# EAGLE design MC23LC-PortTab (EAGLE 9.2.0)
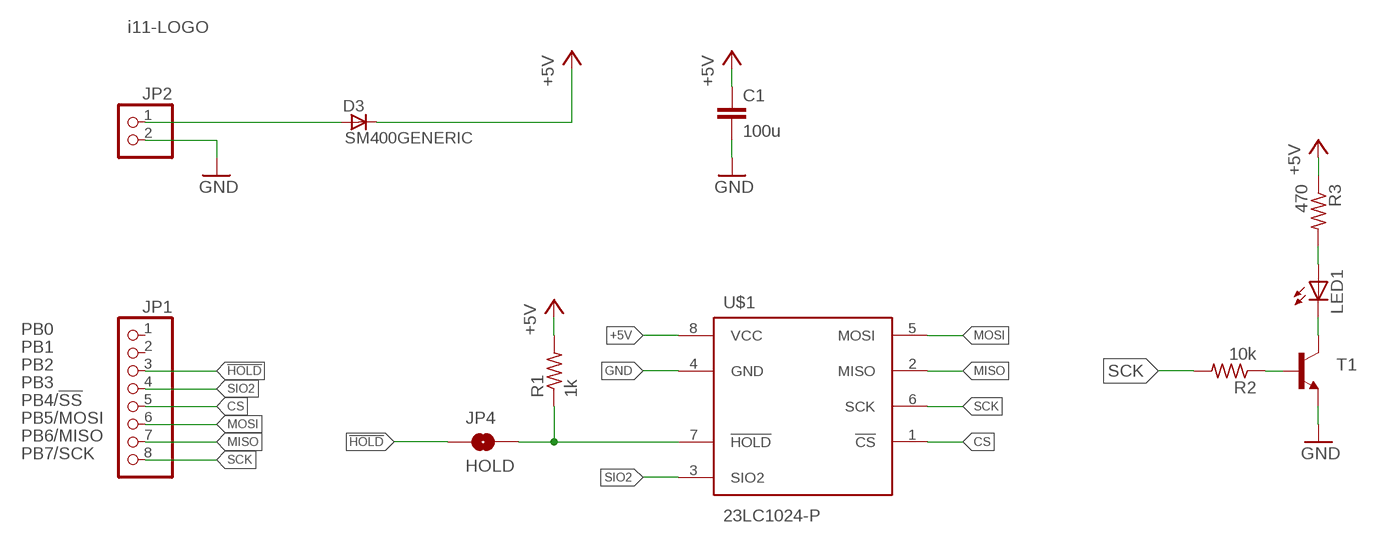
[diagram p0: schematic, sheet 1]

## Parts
C1  100u  C-EUC1206  [C1206]
D3  SM400GENERIC  [MELF-MLL41_DO213AB]
JP1  PINHD-1X8  [1X08]
JP2  PINHD-1X2  [1X02]
JP4  HOLD  JUMPER-SMT_2_NO_SILK  [SMT-JUMPER_2_NO_SILK]
LED1  LEDCHIPLED_1206  [CHIPLED_1206]
R1  1k  R-US_R1206  [R1206]
R2  10k  R-US_R1206  [R1206]
R3  470  R-US_R1206  [R1206]
T1  BC817-16-NPN-SOT23-BEC  [SOT23-BEC]
U$1  23LC1024-P  [DIL8]

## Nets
!HOLD!: JP1.3 JP4.1
+5V: C1.1 D3.C R1.2 R3.1 U$1.8(VCC)
CS: JP1.5 U$1.1(!CS!)
GND: C1.2 JP2.2 T1.E U$1.4(GND)
MISO: JP1.7 U$1.2(MISO)
MOSI: JP1.6 U$1.5(MOSI)
N$1: D3.A JP2.1
N$2: JP4.2 R1.1 U$1.7(!HOLD!)
N$3: R2.1 T1.B
N$5: LED1.C T1.C
N$6: LED1.A R3.2
SCK: JP1.8 R2.2 U$1.6(SCK)
SIO2: JP1.4 U$1.3(SIO2)
Unconnected: JP1.1 JP1.2

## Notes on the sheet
- i11-LOGO
- PB0
- PB1
- PB2
- PB3
- PB4/!SS!
- PB5/MOSI
- PB6/MISO
- PB7/SCK

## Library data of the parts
C1 = rcl:C-EU: CAPACITOR, European symbol; SPICEPREFIX: C
D3 = diodes_smd:SM400*: SM4001 .. SM4007 General Purpose Rectifier, 1 A
JP1 = pinhead:PINHD-1X8: PIN HEADER
JP2 = pinhead:PINHD-1X2: PIN HEADER
JP4 = SparkFun-Jumpers:JUMPER-SMT_2_NO: Normally open jumper
LED1 = led:LED: LED
R1-R3 = rcl:R-US_: RESISTOR, American symbol; SPICEPREFIX: R
T1 = transistor:*-NPN-: NPN Transistror BF959 corrected 2008.03.06
U$1 = MC23LC1024:23LC1024-P

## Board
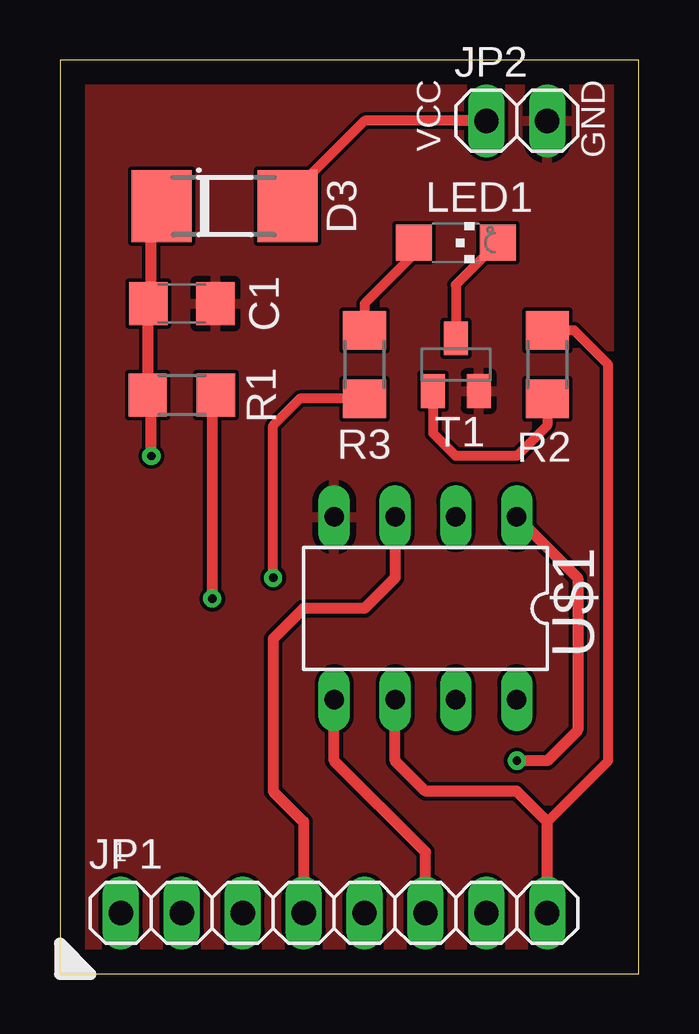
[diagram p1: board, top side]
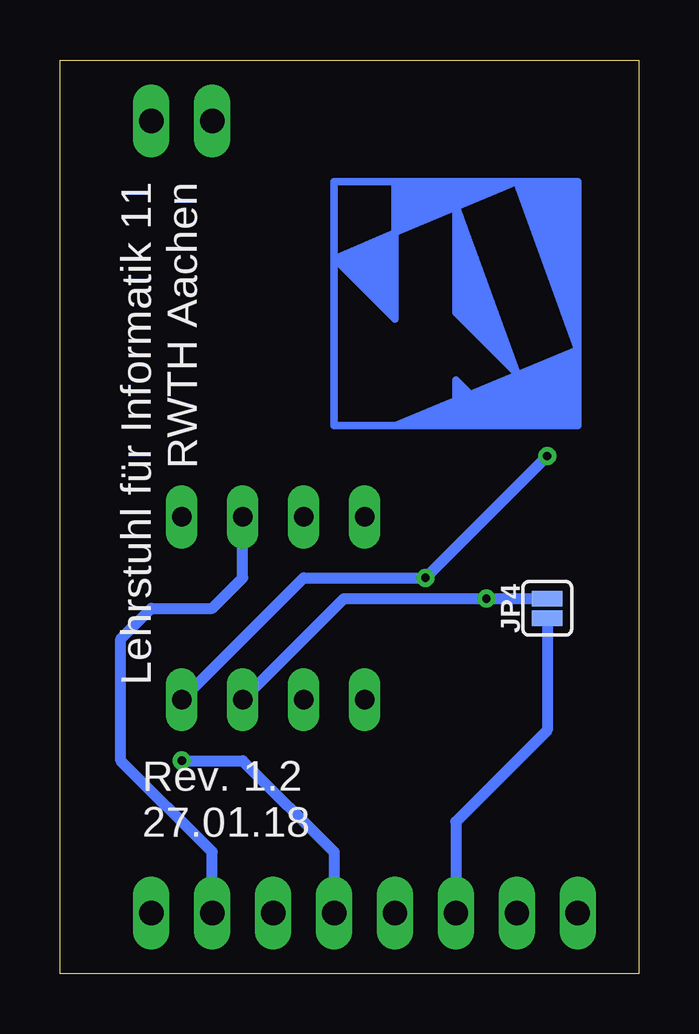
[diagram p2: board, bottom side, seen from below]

Size 24.13 x 38.1 mm. Coordinates in mm from the lower left corner, seen from the top.
Outline: 0,0 24.13,0 24.13,38.1 0,38.1 0,0
Copper layers (1*16): Top 0.035mm / dielectric 1.5mm / Bottom 0.035mm
Design rules "default": minimum track width 6mil, minimum drill 0.35mm, track to track 6mil, track to pad 6mil, pad to pad 6mil, via to via 6mil, smd to smd 6mil, copper to edge 40mil, drill to drill 6mil, minimum pad ring 10mil, minimum via ring 8mil, stop-mask expansion 4mil, vias tented up to drill 0mil, thermal gap 10mil

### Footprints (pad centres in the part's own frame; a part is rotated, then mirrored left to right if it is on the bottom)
C1206 = smd 1.6 x 1.8: 1 -1.4,0; 2 1.4,0
MELF-MLL41_DO213AB = smd 2.5 x 3: A 2.625,0; C -2.625,0
1X08 = drill 1.016 long: 1 -8.89,0; 2 -6.35,0; 3 -3.81,0; 4 -1.27,0; 5 1.27,0; 6 3.81,0; 7 6.35,0; 8 8.89,0
1X02 = drill 1.016 long: 1 -1.27,0; 2 1.27,0
SMT-JUMPER_2_NO_SILK = smd 0.635 x 1.27: 1 -0.406,0; 2 0.406,0
CHIPLED_1206 = smd 1.5 x 1.5: A 0,-1.75; C 0,1.75
R1206 = smd 1.6 x 1.803: 1 -1.422,0; 2 1.422,0
SOT23-BEC = smd 1 x 1.4: B -0.95,-1.1; C 0,1.1; E 0.95,-1.1
DIL8 = drill 0.813 long: 1 -3.81,3.81; 2 -3.81,1.27; 3 -3.81,-1.27; 4 -3.81,-3.81; 5 3.81,-3.81; 6 3.81,-1.27; 7 3.81,1.27; 8 3.81,3.81

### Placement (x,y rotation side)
C1  5.08,27.94 0 top
D3  6.86,32 0 top
JP1  11.43,2.54 0 top
JP2  19.05,35.56 0 top
JP4  3.81,15.24 90 bottom
LED1  16.51,30.48 270 top
R1  5.08,24.13 180 top
R2  20.32,25.4 90 top
R3  12.7,25.4 90 top
T1  16.51,25.4 0 top
U$1  15.24,15.24 270 top
U$2  [LOGO4X4COPPER]  7.62,27.94 0 bottom

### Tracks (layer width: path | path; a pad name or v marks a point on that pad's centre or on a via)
!HOLD!
  Bottom 0.457: JP1.3 7.62,6.35 3.81,10.16 JP4.1
+5V  (via drill 0.35)
  Top 0.406: R3.1 10.01,23.98 8.89,22.86 v8.89,16.51
  Top 0.457: 3.81,23.98 R1.2 3.68,24.15 | 3.68,24.15 C1.1 3.81,28.07 3.81,31.75 4.06,32 D3.C | 3.68,24.15 3.81,24.02 v3.81,21.59
  Bottom 0.457: U$1.8 13.97,16.51 v8.89,16.51 v3.81,21.59
CS  (via drill 0.35)
  Top 0.457: U$1.1 21.59,16.51 21.59,10.16 20.32,8.89 v19.05,8.89
  Bottom 0.457: v19.05,8.89 16.51,8.89 12.7,5.08 JP1.5
GND
  pour Top: 0,38.1 0,0 24.13,0 24.13,38.1
MISO
  Bottom 0.457: JP1.7 17.78,5.08 21.59,8.89 21.59,13.97 20.32,15.24 17.78,15.24 16.51,16.51 U$1.2
MOSI
  Top 0.457: JP1.6 15.24,5.08 11.43,8.89 U$1.5
N$1
  Top 0.406: 16.51,35.56 12.7,35.56 10.16,33.02 10.16,32.68 D3.A
  Top 0.457: JP2.1 16.51,35.56
N$2  (via drill 0.35)
  Top 0.457: R1.1 6.35,23.98 v6.35,15.65
  Bottom 0.457: U$1.7 12.29,15.65 v6.35,15.65 JP4.2
N$3
  Top 0.406: T1.B 15.56,22.54 16.51,21.59 19.05,21.59 20.32,22.86 R2.1
N$5
  Top 0.406: LED1.C 16.51,28.73 T1.C
N$6
  Top 0.406: R3.2 12.7,27.94 14.76,30 LED1.A
SCK
  Top 0.406: 20.32,6.35 22.86,8.89 22.86,25.4 21.44,26.82 R2.2
  Top 0.457: JP1.8 20.32,6.35 19.05,7.62 15.24,7.62 13.97,8.89 U$1.6
SIO2
  Top 0.457: U$1.3 13.97,16.51 12.7,15.24 10.16,15.24 8.89,13.97 8.89,7.62 10.16,6.35 JP1.4

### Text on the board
tNames: VCC | GND | 1
bNames: Lehrstuhl für Informatik 11 / RWTH Aachen | Rev. 1.2 / 27.01.18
